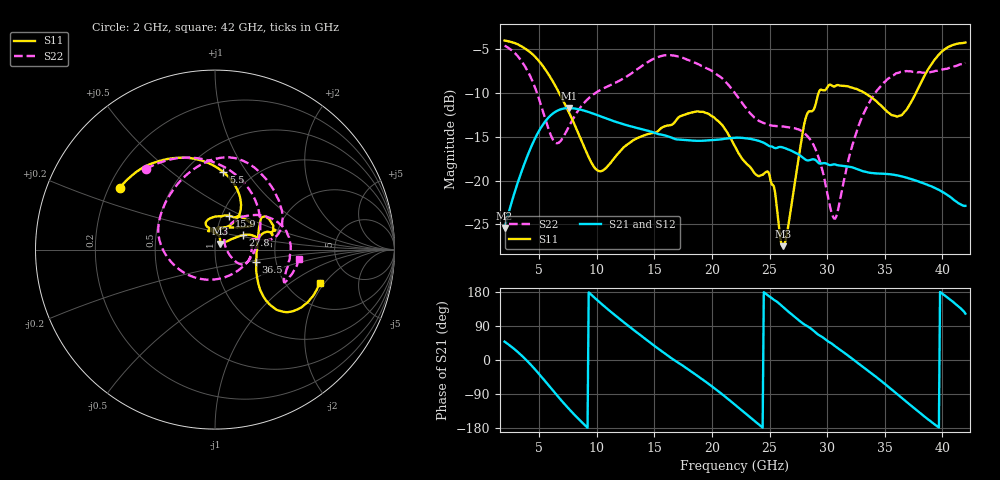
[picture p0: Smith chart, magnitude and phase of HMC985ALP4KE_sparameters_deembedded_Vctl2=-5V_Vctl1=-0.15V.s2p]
!s2p File: Measurements: S11, S21, S12, S22
# GHz S dB R 50.0
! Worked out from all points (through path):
!   401 points, 2 GHz to 42 GHz, reference 50 ohm
!   highest |S21| = -11.71 dB at 7.6 GHz (marker M1); lowest = -25.4 dB at 2 GHz (marker M2)
!   lowest |S11| = -27.5 dB at 26.2 GHz (marker M3), VSWR 1.09, Z = 52.6 + j3.43 ohm
!   |S11| at or under -10 dB: 6.742 GHz to 29.25 GHz (22.51 GHz wide, 125 % of centre); 33.28 GHz to 37.7 GHz (4.42 GHz wide, 12.5 % of centre)
!   |S22| runs from -24.3 to -4.6 dB; largest |S21 - S12| = 0.00025
!   S11 on the Smith chart (normalised r, x): 2 GHz: 0.24, +0.28; 5.5 GHz: 0.74, +0.79; 15.9 GHz: 1.08, +0.43; 27.8 GHz: 1.35, +0.22; 36.5 GHz: 1.57, -0.23; 42 GHz: 3.03, -1.81
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2  -3.98 147.1  -25.43 48.4  -25.44 48.4  -4.57 130.6
3.6  -4.76 120.4  -18.50 8.3  -18.50 8.3  -6.60 85.1
5.5  -7.24 83.9  -13.28 -55.2  -13.29 -55.2  -12.82 2.3
6.5  -9.40 66.8  -12.06 -91.6  -12.07 -91.6  -15.73 -69.8
7.6  -12.25 55.7  -11.71 -129.6  -11.71 -129.6  -13.77 -136.5
8.7  -15.52 57.0  -11.93 -164.1  -11.93 -164.1  -11.43 -170.7
10.2  -18.92 85.9  -12.59 153.7  -12.60 153.7  -9.72 164.9
11.9  -16.84 110.1  -13.39 110.4  -13.40 110.4  -8.63 141.5
15.4  -14.25 76.2  -14.70 28.6  -14.71 28.6  -5.84 87.4
15.9  -13.80 67.7  -14.83 17.5  -14.84 17.5  -5.68 81.2
19.4  -12.23 34.0  -15.44 -56.1  -15.44 -56.0  -7.07 35.6
22  -16.09 51.8  -15.10 -118.1  -15.11 -118.1  -10.00 10.4
24.9  -19.03 103.9  -16.00 169.4  -16.01 169.4  -13.61 13.2
26.2  -27.50 50.4  -16.23 138.9  -16.23 139.0  -13.82 -1.5
27.8  -15.11 27.3  -17.27 98.5  -17.28 98.5  -14.35 -22.8
28.7  -12.06 12.9  -17.57 80.3  -17.58 80.4  -15.62 -29.5
30.7  -9.21 20.9  -18.16 36.2  -18.16 36.2  -24.34 22.5
32.9  -9.74 34.1  -18.84 -13.7  -18.85 -13.7  -13.16 52.7
35.4  -12.30 11.4  -19.27 -72.8  -19.27 -72.8  -8.26 22.0
36.5  -12.49 -16.6  -19.53 -100.6  -19.53 -100.6  -7.53 8.1
39.5  -5.92 -42.8  -20.93 -173.7  -20.93 -173.7  -7.45 -24.8
42  -4.21 -17.5  -22.89 122.4  -22.91 122.4  -6.53 -6.2
